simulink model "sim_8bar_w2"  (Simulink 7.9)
settings: Solver=ode45  StartTime=0.0  StopTime=10  RelTol=1e-3  AbsTol=1e-3
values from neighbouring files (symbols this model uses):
  g = 9806.65    [dyn_2dof.m]    (also in dyn_3dof.m; falling_sphere.m = 9.81; forward_2dof.m = 9.81)
  m = 1    [mechanical_system.m]
  s = Lv/norm(Lv)    [pkm1.m]
undefined symbols (not defined in the file or in its folder): cm, deg, kg, N
libraries: mblibv1 x55

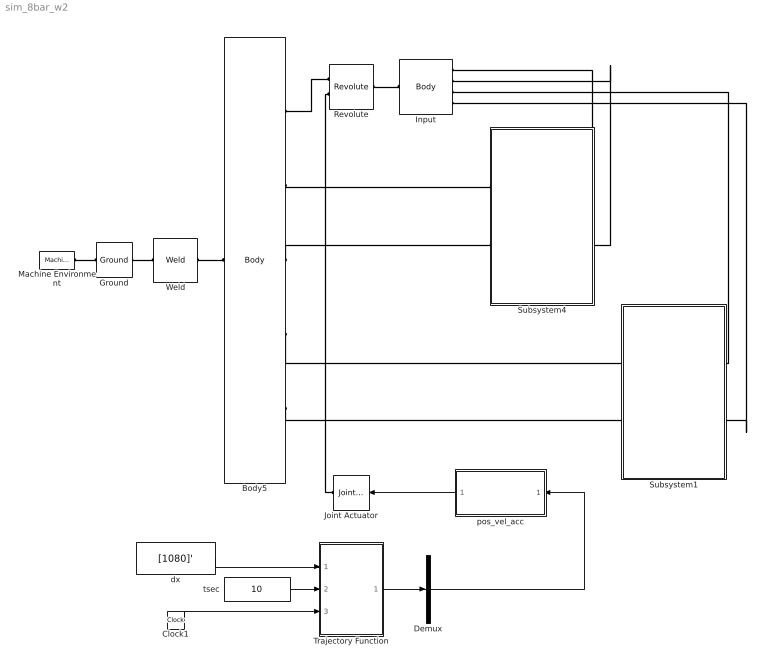
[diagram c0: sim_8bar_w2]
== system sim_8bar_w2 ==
  Body5 : mblibv1/Bodies/Body  LConnTagsString=CS1  RConnTagsString=CS2|CS3|CS4|CS5|CS6  UpdateFromCAD=off  DialogClass=MechanicalBodyBlock  Mass=50  MassUnits=g  InertiaUnits=g*cm^2  Inertia=[0 0 0; 0 0 0; 0 0 0]  Shape=Cylinder  ShapeDims=[1 1]  ShapeUnits=m  ShapeUse=false  Density=1  DensityUnits=kg/m^3  DensityUse=false  GraphicsMode=MACHINE_DEFAULT  BodyColorSelMode=MACHINE_DEFAULT  BodyColor=[1 0 0]  AttachedToCS=CG  CG=Left$CG$[0 0 0]$World$World$mm$[0 0 0]$Euler X-Y-Z$deg$WORLD$false$none  WorkingFrames=Left$CS1$[0 0 0]$World$World$mm$[0 0 0]$Euler X-Y-Z$deg$WORLD$true$none#Right$CS2$[0 0 0]$World$World$mm$[0 0 0]$Euler X-Y-Z$deg$WORLD$true$none#Right$CS3$[-52.5 0 0]$World$World$mm$[0 0 0]$Euler X-Y-Z$deg$WORLD$true$none#Right$CS4$[-52.5 0 0]$World$World$mm$[0 0 0]$Euler X-Y-Z$deg$WORLD$true$none#Right$CS5$[52.5 0 0]$World$World$mm$[0 0 0]$Euler X-Y-Z$deg$WORLD$true$none#Right$CS6$[52.5 0 0]$Worl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  CGPos=[0 0 0]  CGRot=[0 0 0]  CS0Pos=[]  CS0Rot=[]  CS1Pos=[0 0 0]  CS1Rot=[0 0 0]  CS2Pos=[0 0 0]  CS2Rot=[0 0 0]  CS3Pos=[-52.5 0 0]  CS3Rot=[0 0 0]  CS4Pos=[-52.5 0 0]  CS4Rot=[0 0 0]  CS5Pos=[52.5 0 0]  CS5Rot=[0 0 0]  CS6Pos=[52.5 0 0]  CS6Rot=[0 0 0]  CS7Pos=[]  CS7Rot=[]  CS8Pos=[]  CS8Rot=[]  CS9Pos=[]  CS9Rot=[]  CS10Pos=[]  CS10Rot=[]  CS11Pos=[]  CS11Rot=[]  CS12Pos=[]  CS12Rot=[]  CS13Pos=[]  CS13Rot=[]  CS14Pos=[]  CS14Rot=[]  CS15Pos=[]  CS15Rot=[]  CS16Pos=[]  CS16Rot=[]  CS17Pos=[]  CS17Rot=[]  CS18Pos=[]  CS18Rot=[]  CS19Pos=[]  CS19Rot=[]  CS20Pos=[]  CS20Rot=[]
  Clock1 : Clock
  Demux : Demux  Outputs=1
  Ground : mblibv1/Bodies/Ground  UpdateFromCAD=off  LeftPortType=env  RightPortType=workingframe  PhysicalDomain=Mechanical  DialogClass=GroundBlock  CoordPosition=[0 0 0]  CoordPositionUnits=mm  StateVectorMgrId=2  MachineId=[1 0]  ShowEnvPort=on
  Input : mblibv1/Bodies/Body  LConnTagsString=CS1  RConnTagsString=CS2|CS3|CS4|CS5  UpdateFromCAD=off  DialogClass=MechanicalBodyBlock  Mass=1.77  MassUnits=g  InertiaUnits=g*cm^2  Inertia=[1.2556 0 0; 0 1.2556 0; 0 0 0]  Shape=Cylinder  ShapeDims=[1 1]  ShapeUnits=m  ShapeUse=false  Density=1  DensityUnits=kg/m^3  DensityUse=false  GraphicsMode=MACHINE_DEFAULT  BodyColorSelMode=MACHINE_DEFAULT  BodyColor=[1 0 0]  AttachedToCS=CG  CG=Left$CG$[0 7.5 0]$CS1$CS1$mm$[0 0 0]$Euler X-Y-Z$deg$WORLD$false$none  WorkingFrames=Left$CS1$[0 0 0]$World$World$mm$[0 0 0]$Euler X-Y-Z$deg$WORLD$true$none#Right$CS2$[0 15 0]$World$World$mm$[0 0 0]$Euler X-Y-Z$deg$WORLD$true$none#Right$CS3$[0 15 0]$World$World$mm$[0 0 0]$Euler X-Y-Z$deg$WORLD$true$none#Right$CS4$[0 15 0]$World$World$mm$[0 0 0]$Euler X-Y-Z$deg$WORLD$true$none#Right$CS5$[0 15 0]$World$World$mm$[0 0 0]$Euler X-Y-Z$deg$WORLD$true$none  CGPos=[0 7.5 0]  CGRot=[0 0 0]  CS0Pos=[]  CS0Rot=[]  CS1Pos=[0 0 0]  CS1Rot=[0 0 0]  CS2Pos=[0 15 0]  CS2Rot=[0 0 0]  CS3Pos=[0 15 0]  CS3Rot=[0 0 0]  CS4Pos=[0 15 0]  CS4Rot=[0 0 0]  CS5Pos=[0 15 0]  CS5Rot=[0 0 0]  CS6Pos=[]  CS6Rot=[]  CS7Pos=[]  CS7Rot=[]  CS8Pos=[]  CS8Rot=[]  CS9Pos=[]  CS9Rot=[]  CS10Pos=[]  CS10Rot=[]  CS11Pos=[]  CS11Rot=[]  CS12Pos=[]  CS12Rot=[]  CS13Pos=[]  CS13Rot=[]  CS14Pos=[]  CS14Rot=[]  CS15Pos=[]  CS15Rot=[]  CS16Pos=[]  CS16Rot=[]  CS17Pos=[]  CS17Rot=[]  CS18Pos=[]  CS18Rot=[]  CS19Pos=[]  CS19Rot=[]  CS20Pos=[]  CS20Rot=[]
  Joint Actuator : mblibv1/Sensors &  Actuators/Joint Actuator  UpdateFromCAD=off  PhysicalDomain=Mechanical  PortType=blob  ActuationStyle=Motion  AngleUnits=deg  ArcVelocityUnits=deg/s  ArcAccelerationUnits=deg/s^2  CoordPositionUnits=m  VelocityUnits=m/s  AccelerationUnits=m/s^2  ForceUnits=N  TorqueUnits=N*m  ActiveIO=on  Width=3  DialogClass=MechanicalActuatorBlock  Primitive=R1  ReferenceFrame=Absolute (World)
  Machine Environment : mblibv1/Bodies/Machine Environment  PortType=env  PhysicalDomain=Mechanical  DialogTemplateClass=MECH.MachineEnvironment  SyncWhenCopied=off  Gravity=[0 -9.81 0]  GravityUnits=m/s^2  GravityAsSignal=off  Dimensionality=Auto-detect  AnalysisType=Forward dynamics  LinearAssemblyTolerance=1e-3  LinearAssemblyToleranceUnits=m  AngularAssemblyTolerance=1e-3  AngularAssemblyToleranceUnits=rad  ConstraintSolverType=Stabilizing  ConstraintRelTolerance=1e-4  ConstraintAbsTolerance=1e-4  UseRobustSingularityHandling=off  RedundancyAnalysisToleranceType=Automatically select tolerance  RedundancyAnalysisTolerance=1e-14  StatePerturbationType=Fixed  PerturbationSize=1e-5  VisualizeMachine=on  BodyVisualizationType=Use model default body geometries  BodyColorSelMode=Use model default  DefaultBodyColor=[1 0 0]
  Revolute : mblibv1/Joints/Revolute  LConnTagsString=__newl0|SA1  RConnTagsString=__newr0  UpdateFromCAD=off  NumSAPorts=1  CutJoint=off  MarkAsCut=off  Primitives=prismatic  PrimitiveProps=R1$World$[0 0 1]$revolute  DialogClass=JointBlock  R1Axis=[0 0 1]
  Subsystem1 : Subsystem
  Subsystem4 : Subsystem
  Trajectory Function : MATLAB Function  TreatAsAtomicUnit=on
  Weld : mblibv1/Joints/Weld  LConnTagsString=__newl0  RConnTagsString=__newr0  UpdateFromCAD=off  NumSAPorts=0  CutJoint=off  MarkAsCut=off  Primitives=weld  PrimitiveProps=W$WORLD$[0 0 0]$weld  DialogClass=JointBlock  WAxis=[0 0 0]
  dx : Constant  Value=[1080]'
  pos_vel_acc : Subsystem
  tsec : Constant  Value=10
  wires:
  Clock1/1 -> Trajectory Function/3(tout)
  tsec/1 -> Trajectory Function/2(tsec)
  dx/1 -> Trajectory Function/1(dx)
  Demux/1 -> pos_vel_acc/1(In1)
  Trajectory Function/1(xd) -> Demux/1
  pos_vel_acc/1(Motion1) -> Joint Actuator/1
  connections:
  Revolute/RConn1 -- Input/LConn1
  Subsystem4/LConn1 -- Input/RConn1
  Revolute/LConn1 -- Body5/RConn1
  Machine Environment/RConn1 -- Ground/LConn1
  Ground/RConn1 -- Weld/LConn1
  Weld/RConn1 -- Body5/LConn1
  Body5/RConn2 -- Subsystem4/RConn1
  Body5/RConn3 -- Subsystem4/RConn2
  Subsystem4/LConn2 -- Input/RConn2
  Joint Actuator/RConn1 -- Revolute/LConn2
  Body5/RConn4 -- Subsystem1/RConn1
  Body5/RConn5 -- Subsystem1/RConn2
  Input/RConn3 -- Subsystem1/LConn1
  Input/RConn4 -- Subsystem1/LConn2

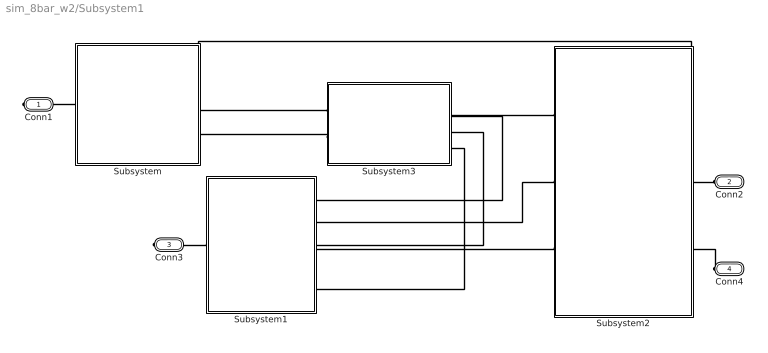
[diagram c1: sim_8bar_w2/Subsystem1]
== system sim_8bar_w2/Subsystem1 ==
  Subsystem : Subsystem
  Subsystem1 : Subsystem
  Subsystem2 : Subsystem
  Subsystem3 : Subsystem
  Conn1 : PMIOPort  Port=1  Side=Right
  Conn2 : PMIOPort  Port=2  Side=Left
  Conn3 : PMIOPort  Port=3  Side=Right
  Conn4 : PMIOPort  Port=4  Side=Left
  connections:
  Subsystem/LConn1 -- Subsystem2/LConn1
  Subsystem/LConn2 -- Subsystem3/LConn1
  Subsystem3/LConn2 -- Subsystem/LConn3
  Subsystem1/LConn1 -- Subsystem3/RConn2
  Subsystem1/LConn2 -- Subsystem2/RConn2
  Subsystem1/LConn3 -- Subsystem3/RConn3
  Subsystem1/LConn4 -- Subsystem2/RConn3
  Subsystem3/RConn4 -- Subsystem1/LConn5
  Subsystem3/RConn1 -- Subsystem2/RConn1
  Conn1/RConn1 -- Subsystem/RConn1
  Conn2/RConn1 -- Subsystem2/LConn2
  Conn3/RConn1 -- Subsystem1/RConn1
  Conn4/RConn1 -- Subsystem2/LConn3

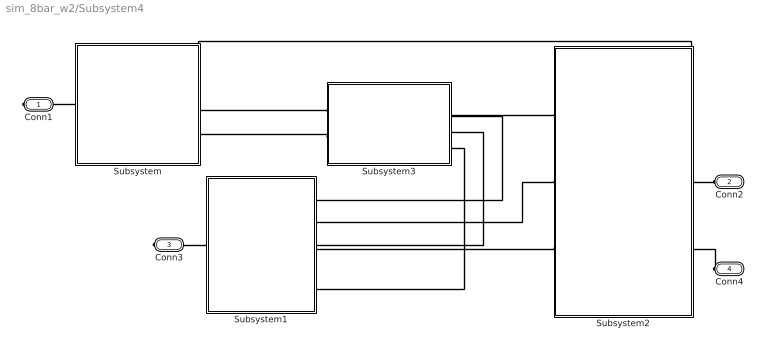
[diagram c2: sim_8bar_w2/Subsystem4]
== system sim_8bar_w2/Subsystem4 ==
  Subsystem : Subsystem
  Subsystem1 : Subsystem
  Subsystem2 : Subsystem
  Subsystem3 : Subsystem
  Conn1 : PMIOPort  Port=1  Side=Right
  Conn2 : PMIOPort  Port=2  Side=Left
  Conn3 : PMIOPort  Port=3  Side=Right
  Conn4 : PMIOPort  Port=4  Side=Left
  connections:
  Subsystem/LConn1 -- Subsystem2/LConn1
  Subsystem/LConn2 -- Subsystem3/LConn1
  Subsystem3/LConn2 -- Subsystem/LConn3
  Subsystem1/LConn1 -- Subsystem3/RConn2
  Subsystem1/LConn2 -- Subsystem2/RConn2
  Subsystem1/LConn3 -- Subsystem3/RConn3
  Subsystem1/LConn4 -- Subsystem2/RConn3
  Subsystem3/RConn4 -- Subsystem1/LConn5
  Subsystem3/RConn1 -- Subsystem2/RConn1
  Conn1/RConn1 -- Subsystem/RConn1
  Conn2/RConn1 -- Subsystem2/LConn2
  Conn3/RConn1 -- Subsystem1/RConn1
  Conn4/RConn1 -- Subsystem2/LConn3

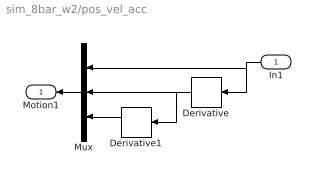
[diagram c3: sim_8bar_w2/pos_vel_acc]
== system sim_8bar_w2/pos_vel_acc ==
  In1 : Inport
  Derivative : Derivative
  Derivative1 : Derivative
  Mux : Mux  Inputs=3
  Motion1 : Outport
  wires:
  Derivative/1 -> Mux/2, Derivative1/1
  Derivative1/1 -> Mux/3
  In1/1 -> Mux/1, Derivative/1
  Mux/1 -> Motion1/1

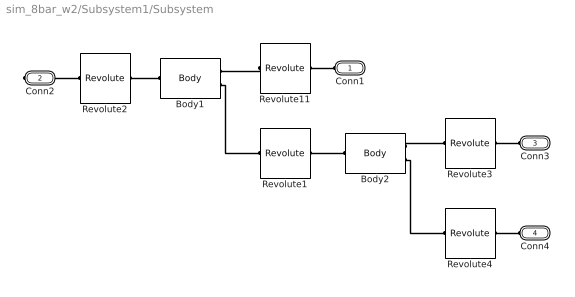
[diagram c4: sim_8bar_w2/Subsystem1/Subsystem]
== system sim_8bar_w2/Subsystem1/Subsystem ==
  Body1 : mblibv1/Bodies/Body  LConnTagsString=CS1  RConnTagsString=CS2|CS3  UpdateFromCAD=off  DialogClass=MechanicalBodyBlock  Mass=4.38  MassUnits=g  InertiaUnits=g*cm^2  Inertia=[4.1121 0 0; 0 4.1121 0; 0 0 0]  Shape=Cylinder  ShapeDims=[1 1]  ShapeUnits=m  ShapeUse=false  Density=1  DensityUnits=kg/m^3  DensityUse=false  GraphicsMode=MACHINE_DEFAULT  BodyColorSelMode=MACHINE_DEFAULT  BodyColor=[1 0 0]  AttachedToCS=CG  CG=Left$CG$[36.37/2 16.21/2 0]$CS1$CS1$mm$[0 0 0]$Euler X-Y-Z$deg$WORLD$false$none  WorkingFrames=Left$CS1$[52.5 0 0]$World$World$mm$[0 0 0]$Euler X-Y-Z$deg$WORLD$true$none#Right$CS2$[64.64 44.37 0]$World$World$mm$[0 0 0]$Euler X-Y-Z$deg$WORLD$true$none#Right$CS3$[96.87 -12.14 0]$World$World$mm$[0 0 0]$Euler X-Y-Z$deg$WORLD$true$none  CGPos=[36.37/2 16.21/2 0]  CGRot=[0 0 0]  CS0Pos=[]  CS0Rot=[]  CS1Pos=[52.5 0 0]  CS1Rot=[0 0 0]  CS2Pos=[64.64 44.37 0]  CS2Rot=[0 0 0]  CS3Pos=[96.87 -12.14 0]  CS3Rot=[0 0 0]  CS4Pos=[]  CS4Rot=[]  CS5Pos=[]  CS5Rot=[]  CS6Pos=[]  CS6Rot=[]  CS7Pos=[]  CS7Rot=[]  CS8Pos=[]  CS8Rot=[]  CS9Pos=[]  CS9Rot=[]  CS10Pos=[]  CS10Rot=[]  CS11Pos=[]  CS11Rot=[]  CS12Pos=[]  CS12Rot=[]  CS13Pos=[]  CS13Rot=[]  CS14Pos=[]  CS14Rot=[]  CS15Pos=[]  CS15Rot=[]  CS16Pos=[]  CS16Rot=[]  CS17Pos=[]  CS17Rot=[]  CS18Pos=[]  CS18Rot=[]  CS19Pos=[]  CS19Rot=[]  CS20Pos=[]  CS20Rot=[]
  Body2 : mblibv1/Bodies/Body  LConnTagsString=CS1  RConnTagsString=CS2|CS3  UpdateFromCAD=off  DialogClass=MechanicalBodyBlock  Mass=2.05  MassUnits=g  InertiaUnits=g*cm^2  Inertia=[1.1579 0 0; 0 1.1579 0; 0 0 0]  Shape=Cylinder  ShapeDims=[1 1]  ShapeUnits=m  ShapeUse=false  Density=1  DensityUnits=kg/m^3  DensityUse=false  GraphicsMode=MACHINE_DEFAULT  BodyColorSelMode=MACHINE_DEFAULT  BodyColor=[1 0 0]  AttachedToCS=CG  CG=Left$CG$[-13.02/2 -43.08/2 0]$CS1$CS1$mm$[0 0 0]$Euler X-Y-Z$deg$WORLD$false$none  WorkingFrames=Left$CS1$[96.87 -12.14 0]$World$World$mm$[0 0 0]$Euler X-Y-Z$deg$WORLD$true$none#Right$CS2$[83.85 -55.22 0]$World$World$mm$[0 0 0]$Euler X-Y-Z$deg$WORLD$true$none#Right$CS3$[83.85 -55.22 0]$World$World$mm$[0 0 0]$Euler X-Y-Z$deg$WORLD$true$none  CGPos=[-13.02/2 -43.08/2 0]  CGRot=[0 0 0]  CS0Pos=[]  CS0Rot=[]  CS1Pos=[96.87 -12.14 0]  CS1Rot=[0 0 0]  CS2Pos=[83.85 -55.22 0]  CS2Rot=[0 0 0]  CS3Pos=[83.85 -55.22 0]  CS3Rot=[0 0 0]  CS4Pos=[]  CS4Rot=[]  CS5Pos=[]  CS5Rot=[]  CS6Pos=[]  CS6Rot=[]  CS7Pos=[]  CS7Rot=[]  CS8Pos=[]  CS8Rot=[]  CS9Pos=[]  CS9Rot=[]  CS10Pos=[]  CS10Rot=[]  CS11Pos=[]  CS11Rot=[]  CS12Pos=[]  CS12Rot=[]  CS13Pos=[]  CS13Rot=[]  CS14Pos=[]  CS14Rot=[]  CS15Pos=[]  CS15Rot=[]  CS16Pos=[]  CS16Rot=[]  CS17Pos=[]  CS17Rot=[]  CS18Pos=[]  CS18Rot=[]  CS19Pos=[]  CS19Rot=[]  CS20Pos=[]  CS20Rot=[]
  Revolute{1..4,11} (5 alike) : mblibv1/Joints/Revolute  LConnTagsString=__newl0  RConnTagsString=__newr0  UpdateFromCAD=off  NumSAPorts=0  CutJoint=off  MarkAsCut=off  Primitives=prismatic  PrimitiveProps=R1$WORLD$[0 0 1]$revolute  DialogClass=JointBlock  R1Axis=[0 0 1]
  Conn1 : PMIOPort  Port=1  Side=Left
  Conn2 : PMIOPort  Port=2  Side=Right
  Conn3 : PMIOPort  Port=3  Side=Left
  Conn4 : PMIOPort  Port=4  Side=Left
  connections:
  Body1/LConn1 -- Revolute2/LConn1
  Revolute11/RConn1 -- Body1/RConn1
  Body1/RConn2 -- Revolute1/RConn1
  Revolute1/LConn1 -- Body2/LConn1
  Body2/RConn1 -- Revolute3/RConn1
  Body2/RConn2 -- Revolute4/RConn1
  Conn1/RConn1 -- Revolute11/LConn1
  Conn2/RConn1 -- Revolute2/RConn1
  Conn3/RConn1 -- Revolute3/LConn1
  Conn4/RConn1 -- Revolute4/LConn1

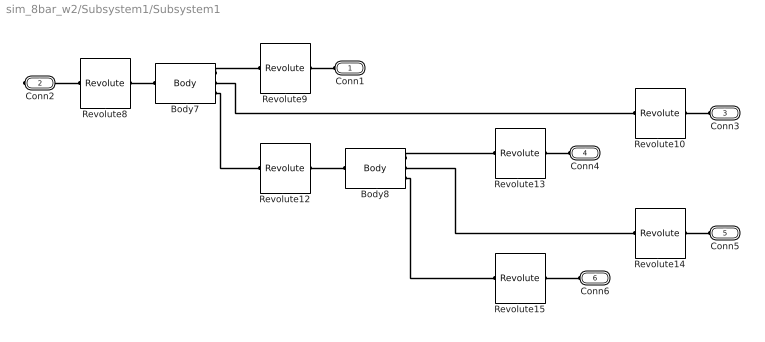
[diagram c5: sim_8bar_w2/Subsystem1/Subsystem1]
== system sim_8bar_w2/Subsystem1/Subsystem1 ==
  Body7 : mblibv1/Bodies/Body  LConnTagsString=CS1  RConnTagsString=CS2|CS3|CS4  UpdateFromCAD=off  DialogClass=MechanicalBodyBlock  Mass=7.25  MassUnits=g  InertiaUnits=g*cm^2  Inertia=[14.8828 0 0; 0 14.8828 0; 0 0 0]  Shape=Cylinder  ShapeDims=[1 1]  ShapeUnits=m  ShapeUse=false  Density=1  DensityUnits=kg/m^3  DensityUse=false  GraphicsMode=MACHINE_DEFAULT  BodyColorSelMode=MACHINE_DEFAULT  BodyColor=[1 0 0]  AttachedToCS=CG  CG=Left$CG$[-12.06/2 -43.55/2 0]$CS1$CS1$mm$[0 0 0]$Euler X-Y-Z$deg$WORLD$false$none  WorkingFrames=Left$CS1$[52.5 0 0]$World$World$mm$[0 0 0]$Euler X-Y-Z$deg$WORLD$true$none#Right$CS2$[40.44 -43.35 0]$World$World$mm$[0 0 0]$Euler X-Y-Z$deg$WORLD$true$none#Right$CS3$[40.44 -43.35 0]$World$World$mm$[0 0 0]$Euler X-Y-Z$deg$WORLD$true$none#Right$CS4$[40.44 -43.35 0]$World$World$mm$[0 0 0]$Euler X-Y-Z$deg$WORLD$true$none  CGPos=[-12.06/2 -43.55/2 0]  CGRot=[0 0 0]  CS0Pos=[]  CS0Rot=[]  CS1Pos=[52.5 0 0]  CS1Rot=[0 0 0]  CS2Pos=[40.44 -43.35 0]  CS2Rot=[0 0 0]  CS3Pos=[40.44 -43.35 0]  CS3Rot=[0 0 0]  CS4Pos=[40.44 -43.35 0]  CS4Rot=[0 0 0]  CS5Pos=[]  CS5Rot=[]  CS6Pos=[]  CS6Rot=[]  CS7Pos=[]  CS7Rot=[]  CS8Pos=[]  CS8Rot=[]  CS9Pos=[]  CS9Rot=[]  CS10Pos=[]  CS10Rot=[]  CS11Pos=[]  CS11Rot=[]  CS12Pos=[]  CS12Rot=[]  CS13Pos=[]  CS13Rot=[]  CS14Pos=[]  CS14Rot=[]  CS15Pos=[]  CS15Rot=[]  CS16Pos=[]  CS16Rot=[]  CS17Pos=[]  CS17Rot=[]  CS18Pos=[]  CS18Rot=[]  CS19Pos=[]  CS19Rot=[]  CS20Pos=[]  CS20Rot=[]
  Body8 : mblibv1/Bodies/Body  LConnTagsString=CS1  RConnTagsString=CS2|CS3|CS4  UpdateFromCAD=off  DialogClass=MechanicalBodyBlock  Mass=9.23  MassUnits=g  InertiaUnits=g*cm^2  Inertia=[7.7797 0 0; 0 7.7797 0; 0 0 0]  Shape=Cylinder  ShapeDims=[1 1]  ShapeUnits=m  ShapeUse=false  Density=1  DensityUnits=kg/m^3  DensityUse=false  GraphicsMode=MACHINE_DEFAULT  BodyColorSelMode=MACHINE_DEFAULT  BodyColor=[1 0 0]  AttachedToCS=CG  CG=Left$CG$[-16.47/2 -57.69/2 0]$CS1$CS1$mm$[0 0 0]$Euler X-Y-Z$deg$WORLD$false$none  WorkingFrames=Left$CS1$[40.44 -43.35 0]$World$World$mm$[0 0 0]$Euler X-Y-Z$deg$WORLD$true$none#Right$CS2$[40.44 -43.35 0]$World$World$mm$[0 0 0]$Euler X-Y-Z$deg$WORLD$true$none#Right$CS3$[40.44 -43.35 0]$World$World$mm$[0 0 0]$Euler X-Y-Z$deg$WORLD$true$none#Right$CS4$[28.09 -86.63 0]$World$World$mm$[0 0 0]$Euler X-Y-Z$deg$WORLD$true$none#Right$CS5$[23.97 -101.05 0]$World$World$mm$[0 0 0]$Euler X-Y-Z$deg$WORLD$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  CGPos=[-16.47/2 -57.69/2 0]  CGRot=[0 0 0]  CS0Pos=[]  CS0Rot=[]  CS1Pos=[40.44 -43.35 0]  CS1Rot=[0 0 0]  CS2Pos=[40.44 -43.35 0]  CS2Rot=[0 0 0]  CS3Pos=[40.44 -43.35 0]  CS3Rot=[0 0 0]  CS4Pos=[28.09 -86.63 0]  CS4Rot=[0 0 0]  CS5Pos=[23.97 -101.05 0]  CS5Rot=[0 0 0]  CS6Pos=[]  CS6Rot=[]  CS7Pos=[]  CS7Rot=[]  CS8Pos=[]  CS8Rot=[]  CS9Pos=[]  CS9Rot=[]  CS10Pos=[]  CS10Rot=[]  CS11Pos=[]  CS11Rot=[]  CS12Pos=[]  CS12Rot=[]  CS13Pos=[]  CS13Rot=[]  CS14Pos=[]  CS14Rot=[]  CS15Pos=[]  CS15Rot=[]  CS16Pos=[]  CS16Rot=[]  CS17Pos=[]  CS17Rot=[]  CS18Pos=[]  CS18Rot=[]  CS19Pos=[]  CS19Rot=[]  CS20Pos=[]  CS20Rot=[]
  Revolute{8..10,12..15} (7 alike) : mblibv1/Joints/Revolute  LConnTagsString=__newl0  RConnTagsString=__newr0  UpdateFromCAD=off  NumSAPorts=0  CutJoint=off  MarkAsCut=off  Primitives=prismatic  PrimitiveProps=R1$WORLD$[0 0 1]$revolute  DialogClass=JointBlock  R1Axis=[0 0 1]
  Conn1 : PMIOPort  Port=1  Side=Left
  Conn2 : PMIOPort  Port=2  Side=Right
  Conn3 : PMIOPort  Port=3  Side=Left
  Conn4 : PMIOPort  Port=4  Side=Left
  Conn5 : PMIOPort  Port=5  Side=Left
  Conn6 : PMIOPort  Port=6  Side=Left
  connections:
  Revolute8/LConn1 -- Body7/LConn1
  Body7/RConn1 -- Revolute9/RConn1
  Body7/RConn2 -- Revolute10/RConn1
  Body7/RConn3 -- Revolute12/RConn1
  Revolute12/LConn1 -- Body8/LConn1
  Body8/RConn1 -- Revolute13/RConn1
  Body8/RConn2 -- Revolute14/RConn1
  Body8/RConn3 -- Revolute15/RConn1
  Conn1/RConn1 -- Revolute9/LConn1
  Conn2/RConn1 -- Revolute8/RConn1
  Conn3/RConn1 -- Revolute10/LConn1
  Conn4/RConn1 -- Revolute13/LConn1
  Conn5/RConn1 -- Revolute14/LConn1
  Conn6/RConn1 -- Revolute15/LConn1

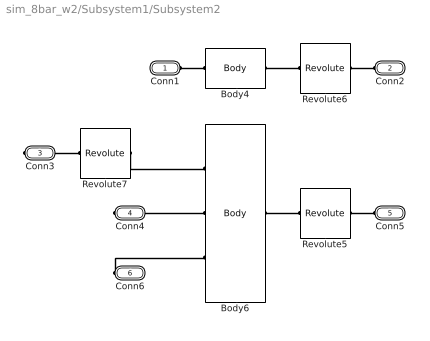
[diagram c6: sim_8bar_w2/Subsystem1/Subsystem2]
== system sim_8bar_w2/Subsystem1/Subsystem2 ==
  Body4 : mblibv1/Bodies/Body  LConnTagsString=CS1  RConnTagsString=CS2  UpdateFromCAD=off  DialogClass=MechanicalBodyBlock  Mass=2.27  MassUnits=g  InertiaUnits=g*cm^2  Inertia=[2.0686 0 0; 0 2.0686 0; 0 0 0]  Shape=Cylinder  ShapeDims=[1 1]  ShapeUnits=m  ShapeUse=false  Density=1  DensityUnits=kg/m^3  DensityUse=false  GraphicsMode=MACHINE_DEFAULT  BodyColorSelMode=MACHINE_DEFAULT  BodyColor=[1 0 0]  AttachedToCS=CG  CG=Left$CG$[-64.64/2 -29.37/2 0]$CS1$CS1$mm$[0 0 0]$Euler X-Y-Z$deg$WORLD$false$none  WorkingFrames=Left$CS1$[64.64 44.37 0]$World$World$mm$[0 0 0]$Euler X-Y-Z$deg$WORLD$true$none#Right$CS2$[0 15 0]$World$World$mm$[0 0 0]$Euler X-Y-Z$deg$WORLD$true$none  CGPos=[-64.64/2 -29.37/2 0]  CGRot=[0 0 0]  CS0Pos=[]  CS0Rot=[]  CS1Pos=[64.64 44.37 0]  CS1Rot=[0 0 0]  CS2Pos=[0 15 0]  CS2Rot=[0 0 0]  CS3Pos=[]  CS3Rot=[]  CS4Pos=[]  CS4Rot=[]  CS5Pos=[]  CS5Rot=[]  CS6Pos=[]  CS6Rot=[]  CS7Pos=[]  CS7Rot=[]  CS8Pos=[]  CS8Rot=[]  CS9Pos=[]  CS9Rot=[]  CS10Pos=[]  CS10Rot=[]  CS11Pos=[]  CS11Rot=[]  CS12Pos=[]  CS12Rot=[]  CS13Pos=[]  CS13Rot=[]  CS14Pos=[]  CS14Rot=[]  CS15Pos=[]  CS15Rot=[]  CS16Pos=[]  CS16Rot=[]  CS17Pos=[]  CS17Rot=[]  CS18Pos=[]  CS18Rot=[]  CS19Pos=[]  CS19Rot=[]  CS20Pos=[]  CS20Rot=[]
  Body6 : mblibv1/Bodies/Body  LConnTagsString=CS1  RConnTagsString=CS2|CS3|CS4  UpdateFromCAD=off  DialogClass=MechanicalBodyBlock  Mass=2.27  MassUnits=g  InertiaUnits=g*cm^2  Inertia=[2.0686 0 0; 0 2.0686 0; 0 0 0]  Shape=Cylinder  ShapeDims=[1 1]  ShapeUnits=m  ShapeUse=false  Density=1  DensityUnits=kg/m^3  DensityUse=false  GraphicsMode=MACHINE_DEFAULT  BodyColorSelMode=MACHINE_DEFAULT  BodyColor=[1 0 0]  AttachedToCS=CG  CG=Left$CG$[40.44/2 -58.35/2 0]$CS1$CS1$mm$[0 0 0]$Euler X-Y-Z$deg$WORLD$false$none  WorkingFrames=Left$CS1$[0 15 0]$World$World$mm$[0 0 0]$Euler X-Y-Z$deg$WORLD$true$none#Right$CS2$[40.44 -43.35 0]$World$World$mm$[0 0 0]$Euler X-Y-Z$deg$WORLD$true$none#Right$CS3$[40.44 -43.35 0]$World$World$mm$[0 0 0]$Euler X-Y-Z$deg$WORLD$true$none#Right$CS4$[40.44 -43.35 0]$World$World$mm$[0 0 0]$Euler X-Y-Z$deg$WORLD$true$none  CGPos=[40.44/2 -58.35/2 0]  CGRot=[0 0 0]  CS0Pos=[]  CS0Rot=[]  CS1Pos=[0 15 0]  CS1Rot=[0 0 0]  CS2Pos=[40.44 -43.35 0]  CS2Rot=[0 0 0]  CS3Pos=[40.44 -43.35 0]  CS3Rot=[0 0 0]  CS4Pos=[40.44 -43.35 0]  CS4Rot=[0 0 0]  CS5Pos=[]  CS5Rot=[]  CS6Pos=[]  CS6Rot=[]  CS7Pos=[]  CS7Rot=[]  CS8Pos=[]  CS8Rot=[]  CS9Pos=[]  CS9Rot=[]  CS10Pos=[]  CS10Rot=[]  CS11Pos=[]  CS11Rot=[]  CS12Pos=[]  CS12Rot=[]  CS13Pos=[]  CS13Rot=[]  CS14Pos=[]  CS14Rot=[]  CS15Pos=[]  CS15Rot=[]  CS16Pos=[]  CS16Rot=[]  CS17Pos=[]  CS17Rot=[]  CS18Pos=[]  CS18Rot=[]  CS19Pos=[]  CS19Rot=[]  CS20Pos=[]  CS20Rot=[]
  Revolute5 : mblibv1/Joints/Revolute  LConnTagsString=__newl0  RConnTagsString=__newr0  UpdateFromCAD=off  NumSAPorts=0  CutJoint=off  MarkAsCut=off  Primitives=prismatic  PrimitiveProps=R1$WORLD$[0 0 1]$revolute  DialogClass=JointBlock  R1Axis=[0 0 1]
  Revolute6 : mblibv1/Joints/Revolute  LConnTagsString=__newl0  RConnTagsString=__newr0  UpdateFromCAD=off  NumSAPorts=0  CutJoint=off  MarkAsCut=off  Primitives=prismatic  PrimitiveProps=R1$WORLD$[0 0 1]$revolute  DialogClass=JointBlock  R1Axis=[0 0 1]
  Revolute7 : mblibv1/Joints/Revolute  LConnTagsString=__newl0  RConnTagsString=__newr0  UpdateFromCAD=off  NumSAPorts=0  CutJoint=off  MarkAsCut=off  Primitives=prismatic  PrimitiveProps=R1$WORLD$[0 0 1]$revolute  DialogClass=JointBlock  R1Axis=[0 0 1]
  Conn1 : PMIOPort  Port=1  Side=Left
  Conn2 : PMIOPort  Port=2  Side=Left
  Conn3 : PMIOPort  Port=3  Side=Right
  Conn4 : PMIOPort  Port=4  Side=Right
  Conn5 : PMIOPort  Port=5  Side=Left
  Conn6 : PMIOPort  Port=6  Side=Right
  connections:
  Body4/RConn1 -- Revolute6/RConn1
  Body6/LConn1 -- Revolute5/RConn1
  Revolute7/LConn1 -- Body6/RConn1
  Conn1/RConn1 -- Body4/LConn1
  Conn2/RConn1 -- Revolute6/LConn1
  Conn3/RConn1 -- Revolute7/RConn1
  Conn4/RConn1 -- Body6/RConn2
  Conn5/RConn1 -- Revolute5/LConn1
  Conn6/RConn1 -- Body6/RConn3

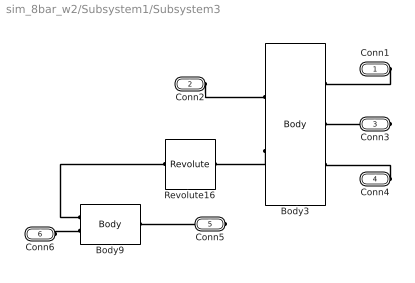
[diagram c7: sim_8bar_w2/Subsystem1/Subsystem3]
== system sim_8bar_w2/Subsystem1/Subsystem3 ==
  Body3 : mblibv1/Bodies/Body  LConnTagsString=CS1|CS5  RConnTagsString=CS2|CS3|CS4  UpdateFromCAD=off  DialogClass=MechanicalBodyBlock  Mass=2.05  MassUnits=g  InertiaUnits=g*cm^2  Inertia=[1.1579 0 0; 0 1.1579 0; 0 0 0]  Shape=Cylinder  ShapeDims=[1 1]  ShapeUnits=m  ShapeUse=false  Density=1  DensityUnits=kg/m^3  DensityUse=false  GraphicsMode=MACHINE_DEFAULT  BodyColorSelMode=MACHINE_DEFAULT  BodyColor=[1 0 0]  AttachedToCS=CG  CG=Left$CG$[-43.41/2 11.86/2 0]$CS1$CS1$mm$[0 0 0]$Euler X-Y-Z$deg$WORLD$false$none  WorkingFrames=Left$CS1$[83.85 -55.22 0]$World$World$mm$[0 0 0]$Euler X-Y-Z$deg$WORLD$true$none#Left$CS5$[83.85 -55.22 0]$World$World$mm$[0 0 0]$Euler X-Y-Z$deg$WORLD$true$none#Right$CS2$[40.44 -43.35 0]$World$World$mm$[0 0 0]$Euler X-Y-Z$deg$WORLD$true$none#Right$CS3$[40.44 -43.35 0]$World$World$mm$[0 0 0]$Euler X-Y-Z$deg$WORLD$true$none#Right$CS4$[40.44 -43.35 0]$World$World$mm$[0 0 0]$Euler X-Y-Z$deg$WORLD$tr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  CGPos=[-43.41/2 11.86/2 0]  CGRot=[0 0 0]  CS0Pos=[]  CS0Rot=[]  CS1Pos=[83.85 -55.22 0]  CS1Rot=[0 0 0]  CS2Pos=[40.44 -43.35 0]  CS2Rot=[0 0 0]  CS3Pos=[40.44 -43.35 0]  CS3Rot=[0 0 0]  CS4Pos=[40.44 -43.35 0]  CS4Rot=[0 0 0]  CS5Pos=[83.85 -55.22 0]  CS5Rot=[0 0 0]  CS6Pos=[]  CS6Rot=[]  CS7Pos=[]  CS7Rot=[]  CS8Pos=[]  CS8Rot=[]  CS9Pos=[]  CS9Rot=[]  CS10Pos=[]  CS10Rot=[]  CS11Pos=[]  CS11Rot=[]  CS12Pos=[]  CS12Rot=[]  CS13Pos=[]  CS13Rot=[]  CS14Pos=[]  CS14Rot=[]  CS15Pos=[]  CS15Rot=[]  CS16Pos=[]  CS16Rot=[]  CS17Pos=[]  CS17Rot=[]  CS18Pos=[]  CS18Rot=[]  CS19Pos=[]  CS19Rot=[]  CS20Pos=[]  CS20Rot=[]
  Body9 : mblibv1/Bodies/Body  LConnTagsString=CS1|CS2  RConnTagsString=CS3  UpdateFromCAD=off  DialogClass=MechanicalBodyBlock  Mass=2.85  MassUnits=g  InertiaUnits=g*cm^2  Inertia=[2.9339 0 0; 0 2.9339 0; 0 0 0]  Shape=Cylinder  ShapeDims=[1 1]  ShapeUnits=m  ShapeUse=false  Density=1  DensityUnits=kg/m^3  DensityUse=false  GraphicsMode=MACHINE_DEFAULT  BodyColorSelMode=MACHINE_DEFAULT  BodyColor=[1 0 0]  AttachedToCS=CG  CG=Left$CG$[-55.76/2 -31.41/2 0]$CS1$CS1$mm$[0 0 0]$Euler X-Y-Z$deg$WORLD$false$none  WorkingFrames=Left$CS1$[83.85 -55.22 0]$World$World$mm$[0 0 0]$Euler X-Y-Z$deg$WORLD$true$none#Left$CS2$[83.85 -55.22 0]$World$World$mm$[0 0 0]$Euler X-Y-Z$deg$WORLD$true$none#Right$CS3$[28.09 -86.63 0]$World$World$mm$[0 0 0]$Euler X-Y-Z$deg$WORLD$true$none  CGPos=[-55.76/2 -31.41/2 0]  CGRot=[0 0 0]  CS0Pos=[]  CS0Rot=[]  CS1Pos=[83.85 -55.22 0]  CS1Rot=[0 0 0]  CS2Pos=[83.85 -55.22 0]  CS2Rot=[0 0 0]  CS3Pos=[28.09 -86.63 0]  CS3Rot=[0 0 0]  CS4Pos=[]  CS4Rot=[]  CS5Pos=[]  CS5Rot=[]  CS6Pos=[]  CS6Rot=[]  CS7Pos=[]  CS7Rot=[]  CS8Pos=[]  CS8Rot=[]  CS9Pos=[]  CS9Rot=[]  CS10Pos=[]  CS10Rot=[]  CS11Pos=[]  CS11Rot=[]  CS12Pos=[]  CS12Rot=[]  CS13Pos=[]  CS13Rot=[]  CS14Pos=[]  CS14Rot=[]  CS15Pos=[]  CS15Rot=[]  CS16Pos=[]  CS16Rot=[]  CS17Pos=[]  CS17Rot=[]  CS18Pos=[]  CS18Rot=[]  CS19Pos=[]  CS19Rot=[]  CS20Pos=[]  CS20Rot=[]
  Revolute16 : mblibv1/Joints/Revolute  LConnTagsString=__newl0  RConnTagsString=__newr0  UpdateFromCAD=off  NumSAPorts=0  CutJoint=off  MarkAsCut=off  Primitives=prismatic  PrimitiveProps=R1$WORLD$[0 0 1]$revolute  DialogClass=JointBlock  R1Axis=[0 0 1]
  Conn1 : PMIOPort  Port=1  Side=Right
  Conn2 : PMIOPort  Port=2  Side=Left
  Conn3 : PMIOPort  Port=3  Side=Right
  Conn4 : PMIOPort  Port=4  Side=Right
  Conn5 : PMIOPort  Port=5  Side=Right
  Conn6 : PMIOPort  Port=6  Side=Left
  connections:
  Body3/LConn2 -- Revolute16/LConn1
  Body9/LConn1 -- Revolute16/RConn1
  Conn1/RConn1 -- Body3/RConn1
  Conn2/RConn1 -- Body3/LConn1
  Conn3/RConn1 -- Body3/RConn2
  Conn4/RConn1 -- Body3/RConn3
  Conn5/RConn1 -- Body9/RConn1
  Conn6/RConn1 -- Body9/LConn2

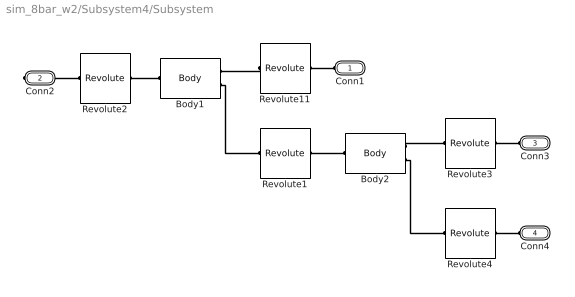
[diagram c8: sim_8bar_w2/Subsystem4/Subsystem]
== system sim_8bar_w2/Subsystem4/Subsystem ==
  Body1 : mblibv1/Bodies/Body  LConnTagsString=CS1  RConnTagsString=CS2|CS3  UpdateFromCAD=off  DialogClass=MechanicalBodyBlock  Mass=4.38  MassUnits=g  InertiaUnits=g*cm^2  Inertia=[4.1121 0 0; 0 4.1121 0; 0 0 0]  Shape=Cylinder  ShapeDims=[1 1]  ShapeUnits=m  ShapeUse=false  Density=1  DensityUnits=kg/m^3  DensityUse=false  GraphicsMode=MACHINE_DEFAULT  BodyColorSelMode=MACHINE_DEFAULT  BodyColor=[1 0 0]  AttachedToCS=CG  CG=Left$CG$[-36.37/2 16.21/2 0]$CS1$CS1$mm$[0 0 0]$Euler X-Y-Z$deg$WORLD$false$none  WorkingFrames=Left$CS1$[-52.5 0 0]$World$World$mm$[0 0 0]$Euler X-Y-Z$deg$WORLD$true$none#Right$CS2$[-64.64 44.37 0]$World$World$mm$[0 0 0]$Euler X-Y-Z$deg$WORLD$true$none#Right$CS3$[-96.87 -12.14 0]$World$World$mm$[0 0 0]$Euler X-Y-Z$deg$WORLD$true$none  CGPos=[-36.37/2 16.21/2 0]  CGRot=[0 0 0]  CS0Pos=[]  CS0Rot=[]  CS1Pos=[-52.5 0 0]  CS1Rot=[0 0 0]  CS2Pos=[-64.64 44.37 0]  CS2Rot=[0 0 0]  CS3Pos=[-96.87 -12.14 0]  CS3Rot=[0 0 0]  CS4Pos=[]  CS4Rot=[]  CS5Pos=[]  CS5Rot=[]  CS6Pos=[]  CS6Rot=[]  CS7Pos=[]  CS7Rot=[]  CS8Pos=[]  CS8Rot=[]  CS9Pos=[]  CS9Rot=[]  CS10Pos=[]  CS10Rot=[]  CS11Pos=[]  CS11Rot=[]  CS12Pos=[]  CS12Rot=[]  CS13Pos=[]  CS13Rot=[]  CS14Pos=[]  CS14Rot=[]  CS15Pos=[]  CS15Rot=[]  CS16Pos=[]  CS16Rot=[]  CS17Pos=[]  CS17Rot=[]  CS18Pos=[]  CS18Rot=[]  CS19Pos=[]  CS19Rot=[]  CS20Pos=[]  CS20Rot=[]
  Body2 : mblibv1/Bodies/Body  LConnTagsString=CS1  RConnTagsString=CS2|CS3  UpdateFromCAD=off  DialogClass=MechanicalBodyBlock  Mass=2.05  MassUnits=g  InertiaUnits=g*cm^2  Inertia=[1.1579 0 0; 0 1.1579 0; 0 0 0]  Shape=Cylinder  ShapeDims=[1 1]  ShapeUnits=m  ShapeUse=false  Density=1  DensityUnits=kg/m^3  DensityUse=false  GraphicsMode=MACHINE_DEFAULT  BodyColorSelMode=MACHINE_DEFAULT  BodyColor=[1 0 0]  AttachedToCS=CG  CG=Left$CG$[13.02/2 -43.08/2 0]$CS1$CS1$mm$[0 0 0]$Euler X-Y-Z$deg$WORLD$false$none  WorkingFrames=Left$CS1$[-96.87 -12.14 0]$World$World$mm$[0 0 0]$Euler X-Y-Z$deg$WORLD$true$none#Right$CS2$[-83.85 -55.22 0]$World$World$mm$[0 0 0]$Euler X-Y-Z$deg$WORLD$true$none#Right$CS3$[-83.85 -55.22 0]$World$World$mm$[0 0 0]$Euler X-Y-Z$deg$WORLD$true$none  CGPos=[13.02/2 -43.08/2 0]  CGRot=[0 0 0]  CS0Pos=[]  CS0Rot=[]  CS1Pos=[-96.87 -12.14 0]  CS1Rot=[0 0 0]  CS2Pos=[-83.85 -55.22 0]  CS2Rot=[0 0 0]  CS3Pos=[-83.85 -55.22 0]  CS3Rot=[0 0 0]  CS4Pos=[]  CS4Rot=[]  CS5Pos=[]  CS5Rot=[]  CS6Pos=[]  CS6Rot=[]  CS7Pos=[]  CS7Rot=[]  CS8Pos=[]  CS8Rot=[]  CS9Pos=[]  CS9Rot=[]  CS10Pos=[]  CS10Rot=[]  CS11Pos=[]  CS11Rot=[]  CS12Pos=[]  CS12Rot=[]  CS13Pos=[]  CS13Rot=[]  CS14Pos=[]  CS14Rot=[]  CS15Pos=[]  CS15Rot=[]  CS16Pos=[]  CS16Rot=[]  CS17Pos=[]  CS17Rot=[]  CS18Pos=[]  CS18Rot=[]  CS19Pos=[]  CS19Rot=[]  CS20Pos=[]  CS20Rot=[]
  Revolute{1..4,11} (5 alike) : mblibv1/Joints/Revolute  LConnTagsString=__newl0  RConnTagsString=__newr0  UpdateFromCAD=off  NumSAPorts=0  CutJoint=off  MarkAsCut=off  Primitives=prismatic  PrimitiveProps=R1$WORLD$[0 0 1]$revolute  DialogClass=JointBlock  R1Axis=[0 0 1]
  Conn1 : PMIOPort  Port=1  Side=Left
  Conn2 : PMIOPort  Port=2  Side=Right
  Conn3 : PMIOPort  Port=3  Side=Left
  Conn4 : PMIOPort  Port=4  Side=Left
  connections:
  Body1/LConn1 -- Revolute2/LConn1
  Revolute11/RConn1 -- Body1/RConn1
  Body1/RConn2 -- Revolute1/RConn1
  Revolute1/LConn1 -- Body2/LConn1
  Body2/RConn1 -- Revolute3/RConn1
  Body2/RConn2 -- Revolute4/RConn1
  Conn1/RConn1 -- Revolute11/LConn1
  Conn2/RConn1 -- Revolute2/RConn1
  Conn3/RConn1 -- Revolute3/LConn1
  Conn4/RConn1 -- Revolute4/LConn1

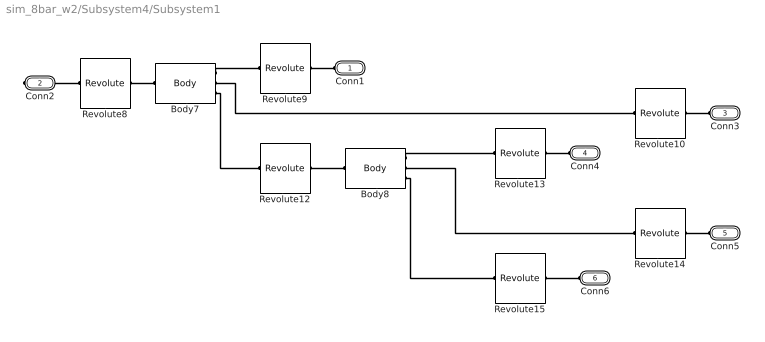
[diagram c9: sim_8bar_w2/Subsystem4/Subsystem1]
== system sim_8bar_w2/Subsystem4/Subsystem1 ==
  Body7 : mblibv1/Bodies/Body  LConnTagsString=CS1  RConnTagsString=CS2|CS3|CS4  UpdateFromCAD=off  DialogClass=MechanicalBodyBlock  Mass=7.25  MassUnits=g  InertiaUnits=g*cm^2  Inertia=[14.8828 0 0; 0 14.8828 0; 0 0 0]  Shape=Cylinder  ShapeDims=[1 1]  ShapeUnits=m  ShapeUse=false  Density=1  DensityUnits=kg/m^3  DensityUse=false  GraphicsMode=MACHINE_DEFAULT  BodyColorSelMode=MACHINE_DEFAULT  BodyColor=[1 0 0]  AttachedToCS=CG  CG=Left$CG$[12.06/2 -43.55/2 0]$CS1$CS1$mm$[0 0 0]$Euler X-Y-Z$deg$WORLD$false$none  WorkingFrames=Left$CS1$[-52.5 0 0]$World$World$mm$[0 0 0]$Euler X-Y-Z$deg$WORLD$true$none#Right$CS2$[-40.44 -43.35 0]$World$World$mm$[0 0 0]$Euler X-Y-Z$deg$WORLD$true$none#Right$CS3$[-40.44 -43.35 0]$World$World$mm$[0 0 0]$Euler X-Y-Z$deg$WORLD$true$none#Right$CS4$[-40.44 -43.35 0]$World$World$mm$[0 0 0]$Euler X-Y-Z$deg$WORLD$true$none  CGPos=[12.06/2 -43.55/2 0]  CGRot=[0 0 0]  CS0Pos=[]  CS0Rot=[]  CS1Pos=[-52.5 0 0]  CS1Rot=[0 0 0]  CS2Pos=[-40.44 -43.35 0]  CS2Rot=[0 0 0]  CS3Pos=[-40.44 -43.35 0]  CS3Rot=[0 0 0]  CS4Pos=[-40.44 -43.35 0]  CS4Rot=[0 0 0]  CS5Pos=[]  CS5Rot=[]  CS6Pos=[]  CS6Rot=[]  CS7Pos=[]  CS7Rot=[]  CS8Pos=[]  CS8Rot=[]  CS9Pos=[]  CS9Rot=[]  CS10Pos=[]  CS10Rot=[]  CS11Pos=[]  CS11Rot=[]  CS12Pos=[]  CS12Rot=[]  CS13Pos=[]  CS13Rot=[]  CS14Pos=[]  CS14Rot=[]  CS15Pos=[]  CS15Rot=[]  CS16Pos=[]  CS16Rot=[]  CS17Pos=[]  CS17Rot=[]  CS18Pos=[]  CS18Rot=[]  CS19Pos=[]  CS19Rot=[]  CS20Pos=[]  CS20Rot=[]
  Body8 : mblibv1/Bodies/Body  LConnTagsString=CS1  RConnTagsString=CS2|CS3|CS4  UpdateFromCAD=off  DialogClass=MechanicalBodyBlock  Mass=9.23  MassUnits=g  InertiaUnits=g*cm^2  Inertia=[7.7797 0 0; 0 7.7797 0; 0 0 0]  Shape=Cylinder  ShapeDims=[1 1]  ShapeUnits=m  ShapeUse=false  Density=1  DensityUnits=kg/m^3  DensityUse=false  GraphicsMode=MACHINE_DEFAULT  BodyColorSelMode=MACHINE_DEFAULT  BodyColor=[1 0 0]  AttachedToCS=CG  CG=Left$CG$[16.47/2 -57.69/2 0]$CS1$CS1$mm$[0 0 0]$Euler X-Y-Z$deg$WORLD$false$none  WorkingFrames=Left$CS1$[-40.44 -43.35 0]$World$World$mm$[0 0 0]$Euler X-Y-Z$deg$WORLD$true$none#Right$CS2$[-40.44 -43.35 0]$World$World$mm$[0 0 0]$Euler X-Y-Z$deg$WORLD$true$none#Right$CS3$[-40.44 -43.35 0]$World$World$mm$[0 0 0]$Euler X-Y-Z$deg$WORLD$true$none#Right$CS4$[-28.09 -86.63 0]$World$World$mm$[0 0 0]$Euler X-Y-Z$deg$WORLD$true$none#Right$CS5$[-23.97 -101.05 0]$World$World$mm$[0 0 0]$Euler X-Y-Z$deg$W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  CGPos=[16.47/2 -57.69/2 0]  CGRot=[0 0 0]  CS0Pos=[]  CS0Rot=[]  CS1Pos=[-40.44 -43.35 0]  CS1Rot=[0 0 0]  CS2Pos=[-40.44 -43.35 0]  CS2Rot=[0 0 0]  CS3Pos=[-40.44 -43.35 0]  CS3Rot=[0 0 0]  CS4Pos=[-28.09 -86.63 0]  CS4Rot=[0 0 0]  CS5Pos=[-23.97 -101.05 0]  CS5Rot=[0 0 0]  CS6Pos=[]  CS6Rot=[]  CS7Pos=[]  CS7Rot=[]  CS8Pos=[]  CS8Rot=[]  CS9Pos=[]  CS9Rot=[]  CS10Pos=[]  CS10Rot=[]  CS11Pos=[]  CS11Rot=[]  CS12Pos=[]  CS12Rot=[]  CS13Pos=[]  CS13Rot=[]  CS14Pos=[]  CS14Rot=[]  CS15Pos=[]  CS15Rot=[]  CS16Pos=[]  CS16Rot=[]  CS17Pos=[]  CS17Rot=[]  CS18Pos=[]  CS18Rot=[]  CS19Pos=[]  CS19Rot=[]  CS20Pos=[]  CS20Rot=[]
  Revolute{8..10,12..15} (7 alike) : mblibv1/Joints/Revolute  LConnTagsString=__newl0  RConnTagsString=__newr0  UpdateFromCAD=off  NumSAPorts=0  CutJoint=off  MarkAsCut=off  Primitives=prismatic  PrimitiveProps=R1$WORLD$[0 0 1]$revolute  DialogClass=JointBlock  R1Axis=[0 0 1]
  Conn1 : PMIOPort  Port=1  Side=Left
  Conn2 : PMIOPort  Port=2  Side=Right
  Conn3 : PMIOPort  Port=3  Side=Left
  Conn4 : PMIOPort  Port=4  Side=Left
  Conn5 : PMIOPort  Port=5  Side=Left
  Conn6 : PMIOPort  Port=6  Side=Left
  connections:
  Revolute8/LConn1 -- Body7/LConn1
  Body7/RConn1 -- Revolute9/RConn1
  Body7/RConn2 -- Revolute10/RConn1
  Body7/RConn3 -- Revolute12/RConn1
  Revolute12/LConn1 -- Body8/LConn1
  Body8/RConn1 -- Revolute13/RConn1
  Body8/RConn2 -- Revolute14/RConn1
  Body8/RConn3 -- Revolute15/RConn1
  Conn1/RConn1 -- Revolute9/LConn1
  Conn2/RConn1 -- Revolute8/RConn1
  Conn3/RConn1 -- Revolute10/LConn1
  Conn4/RConn1 -- Revolute13/LConn1
  Conn5/RConn1 -- Revolute14/LConn1
  Conn6/RConn1 -- Revolute15/LConn1

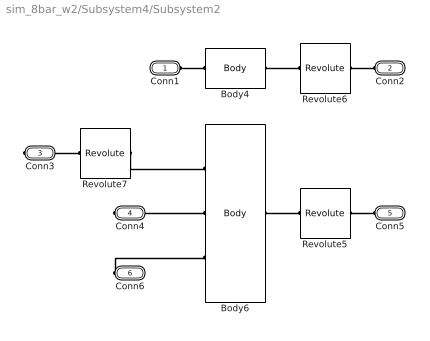
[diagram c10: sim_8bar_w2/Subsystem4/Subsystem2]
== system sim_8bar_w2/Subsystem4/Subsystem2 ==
  Body4 : mblibv1/Bodies/Body  LConnTagsString=CS1  RConnTagsString=CS2  UpdateFromCAD=off  DialogClass=MechanicalBodyBlock  Mass=2.27  MassUnits=g  InertiaUnits=g*cm^2  Inertia=[2.0686 0 0; 0 2.0686 0; 0 0 0]  Shape=Cylinder  ShapeDims=[1 1]  ShapeUnits=m  ShapeUse=false  Density=1  DensityUnits=kg/m^3  DensityUse=false  GraphicsMode=MACHINE_DEFAULT  BodyColorSelMode=MACHINE_DEFAULT  BodyColor=[1 0 0]  AttachedToCS=CG  CG=Left$CG$[64.64/2 -29.37/2 0]$CS1$CS1$mm$[0 0 0]$Euler X-Y-Z$deg$WORLD$false$none  WorkingFrames=Left$CS1$[-64.64 44.37 0]$World$World$mm$[0 0 0]$Euler X-Y-Z$deg$WORLD$true$none#Right$CS2$[0 15 0]$World$World$mm$[0 0 0]$Euler X-Y-Z$deg$WORLD$true$none  CGPos=[64.64/2 -29.37/2 0]  CGRot=[0 0 0]  CS0Pos=[]  CS0Rot=[]  CS1Pos=[-64.64 44.37 0]  CS1Rot=[0 0 0]  CS2Pos=[0 15 0]  CS2Rot=[0 0 0]  CS3Pos=[]  CS3Rot=[]  CS4Pos=[]  CS4Rot=[]  CS5Pos=[]  CS5Rot=[]  CS6Pos=[]  CS6Rot=[]  CS7Pos=[]  CS7Rot=[]  CS8Pos=[]  CS8Rot=[]  CS9Pos=[]  CS9Rot=[]  CS10Pos=[]  CS10Rot=[]  CS11Pos=[]  CS11Rot=[]  CS12Pos=[]  CS12Rot=[]  CS13Pos=[]  CS13Rot=[]  CS14Pos=[]  CS14Rot=[]  CS15Pos=[]  CS15Rot=[]  CS16Pos=[]  CS16Rot=[]  CS17Pos=[]  CS17Rot=[]  CS18Pos=[]  CS18Rot=[]  CS19Pos=[]  CS19Rot=[]  CS20Pos=[]  CS20Rot=[]
  Body6 : mblibv1/Bodies/Body  LConnTagsString=CS1  RConnTagsString=CS2|CS3|CS4  UpdateFromCAD=off  DialogClass=MechanicalBodyBlock  Mass=2.27  MassUnits=g  InertiaUnits=g*cm^2  Inertia=[2.0686 0 0; 0 2.0686 0; 0 0 0]  Shape=Cylinder  ShapeDims=[1 1]  ShapeUnits=m  ShapeUse=false  Density=1  DensityUnits=kg/m^3  DensityUse=false  GraphicsMode=MACHINE_DEFAULT  BodyColorSelMode=MACHINE_DEFAULT  BodyColor=[1 0 0]  AttachedToCS=CG  CG=Left$CG$[-40.44/2 -58.35/2 0]$CS1$CS1$mm$[0 0 0]$Euler X-Y-Z$deg$WORLD$false$none  WorkingFrames=Left$CS1$[0 15 0]$World$World$mm$[0 0 0]$Euler X-Y-Z$deg$WORLD$true$none#Right$CS2$[-40.44 -43.35 0]$World$World$mm$[0 0 0]$Euler X-Y-Z$deg$WORLD$true$none#Right$CS3$[-40.44 -43.35 0]$World$World$mm$[0 0 0]$Euler X-Y-Z$deg$WORLD$true$none#Right$CS4$[-40.44 -43.35 0]$World$World$mm$[0 0 0]$Euler X-Y-Z$deg$WORLD$true$none  CGPos=[-40.44/2 -58.35/2 0]  CGRot=[0 0 0]  CS0Pos=[]  CS0Rot=[]  CS1Pos=[0 15 0]  CS1Rot=[0 0 0]  CS2Pos=[-40.44 -43.35 0]  CS2Rot=[0 0 0]  CS3Pos=[-40.44 -43.35 0]  CS3Rot=[0 0 0]  CS4Pos=[-40.44 -43.35 0]  CS4Rot=[0 0 0]  CS5Pos=[]  CS5Rot=[]  CS6Pos=[]  CS6Rot=[]  CS7Pos=[]  CS7Rot=[]  CS8Pos=[]  CS8Rot=[]  CS9Pos=[]  CS9Rot=[]  CS10Pos=[]  CS10Rot=[]  CS11Pos=[]  CS11Rot=[]  CS12Pos=[]  CS12Rot=[]  CS13Pos=[]  CS13Rot=[]  CS14Pos=[]  CS14Rot=[]  CS15Pos=[]  CS15Rot=[]  CS16Pos=[]  CS16Rot=[]  CS17Pos=[]  CS17Rot=[]  CS18Pos=[]  CS18Rot=[]  CS19Pos=[]  CS19Rot=[]  CS20Pos=[]  CS20Rot=[]
  Revolute5 : mblibv1/Joints/Revolute  LConnTagsString=__newl0  RConnTagsString=__newr0  UpdateFromCAD=off  NumSAPorts=0  CutJoint=off  MarkAsCut=off  Primitives=prismatic  PrimitiveProps=R1$WORLD$[0 0 1]$revolute  DialogClass=JointBlock  R1Axis=[0 0 1]
  Revolute6 : mblibv1/Joints/Revolute  LConnTagsString=__newl0  RConnTagsString=__newr0  UpdateFromCAD=off  NumSAPorts=0  CutJoint=off  MarkAsCut=off  Primitives=prismatic  PrimitiveProps=R1$WORLD$[0 0 1]$revolute  DialogClass=JointBlock  R1Axis=[0 0 1]
  Revolute7 : mblibv1/Joints/Revolute  LConnTagsString=__newl0  RConnTagsString=__newr0  UpdateFromCAD=off  NumSAPorts=0  CutJoint=off  MarkAsCut=off  Primitives=prismatic  PrimitiveProps=R1$WORLD$[0 0 1]$revolute  DialogClass=JointBlock  R1Axis=[0 0 1]
  Conn1 : PMIOPort  Port=1  Side=Left
  Conn2 : PMIOPort  Port=2  Side=Left
  Conn3 : PMIOPort  Port=3  Side=Right
  Conn4 : PMIOPort  Port=4  Side=Right
  Conn5 : PMIOPort  Port=5  Side=Left
  Conn6 : PMIOPort  Port=6  Side=Right
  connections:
  Body4/RConn1 -- Revolute6/RConn1
  Body6/LConn1 -- Revolute5/RConn1
  Revolute7/LConn1 -- Body6/RConn1
  Conn1/RConn1 -- Body4/LConn1
  Conn2/RConn1 -- Revolute6/LConn1
  Conn3/RConn1 -- Revolute7/RConn1
  Conn4/RConn1 -- Body6/RConn2
  Conn5/RConn1 -- Revolute5/LConn1
  Conn6/RConn1 -- Body6/RConn3

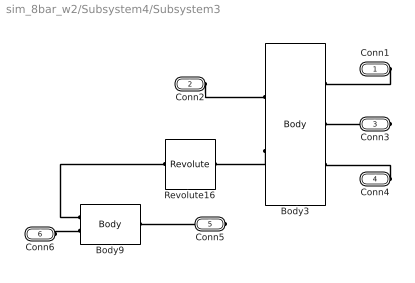
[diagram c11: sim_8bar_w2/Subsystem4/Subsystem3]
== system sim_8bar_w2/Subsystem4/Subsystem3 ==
  Body3 : mblibv1/Bodies/Body  LConnTagsString=CS1|CS5  RConnTagsString=CS2|CS3|CS4  UpdateFromCAD=off  DialogClass=MechanicalBodyBlock  Mass=2.05  MassUnits=g  InertiaUnits=g*cm^2  Inertia=[1.1579 0 0; 0 1.1579 0; 0 0 0]  Shape=Cylinder  ShapeDims=[1 1]  ShapeUnits=m  ShapeUse=false  Density=1  DensityUnits=kg/m^3  DensityUse=false  GraphicsMode=MACHINE_DEFAULT  BodyColorSelMode=MACHINE_DEFAULT  BodyColor=[1 0 0]  AttachedToCS=CG  CG=Left$CG$[43.41/2 11.86/2 0]$CS1$CS1$mm$[0 0 0]$Euler X-Y-Z$deg$WORLD$false$none  WorkingFrames=Left$CS1$[-83.85 -55.22 0]$World$World$mm$[0 0 0]$Euler X-Y-Z$deg$WORLD$true$none#Left$CS5$[-83.85 -55.22 0]$World$World$mm$[0 0 0]$Euler X-Y-Z$deg$WORLD$true$none#Right$CS2$[-40.44 -43.35 0]$World$World$mm$[0 0 0]$Euler X-Y-Z$deg$WORLD$true$none#Right$CS3$[-40.44 -43.35 0]$World$World$mm$[0 0 0]$Euler X-Y-Z$deg$WORLD$true$none#Right$CS4$[-40.44 -43.35 0]$World$World$mm$[0 0 0]$Euler X-Y-Z$deg$WOR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  CGPos=[43.41/2 11.86/2 0]  CGRot=[0 0 0]  CS0Pos=[]  CS0Rot=[]  CS1Pos=[-83.85 -55.22 0]  CS1Rot=[0 0 0]  CS2Pos=[-40.44 -43.35 0]  CS2Rot=[0 0 0]  CS3Pos=[-40.44 -43.35 0]  CS3Rot=[0 0 0]  CS4Pos=[-40.44 -43.35 0]  CS4Rot=[0 0 0]  CS5Pos=[-83.85 -55.22 0]  CS5Rot=[0 0 0]  CS6Pos=[]  CS6Rot=[]  CS7Pos=[]  CS7Rot=[]  CS8Pos=[]  CS8Rot=[]  CS9Pos=[]  CS9Rot=[]  CS10Pos=[]  CS10Rot=[]  CS11Pos=[]  CS11Rot=[]  CS12Pos=[]  CS12Rot=[]  CS13Pos=[]  CS13Rot=[]  CS14Pos=[]  CS14Rot=[]  CS15Pos=[]  CS15Rot=[]  CS16Pos=[]  CS16Rot=[]  CS17Pos=[]  CS17Rot=[]  CS18Pos=[]  CS18Rot=[]  CS19Pos=[]  CS19Rot=[]  CS20Pos=[]  CS20Rot=[]
  Body9 : mblibv1/Bodies/Body  LConnTagsString=CS1|CS2  RConnTagsString=CS3  UpdateFromCAD=off  DialogClass=MechanicalBodyBlock  Mass=2.85  MassUnits=g  InertiaUnits=g*cm^2  Inertia=[2.9339 0 0; 0 2.9339 0; 0 0 0]  Shape=Cylinder  ShapeDims=[1 1]  ShapeUnits=m  ShapeUse=false  Density=1  DensityUnits=kg/m^3  DensityUse=false  GraphicsMode=MACHINE_DEFAULT  BodyColorSelMode=MACHINE_DEFAULT  BodyColor=[1 0 0]  AttachedToCS=CG  CG=Left$CG$[55.76/2 -31.41/2 0]$CS1$CS1$mm$[0 0 0]$Euler X-Y-Z$deg$WORLD$false$none  WorkingFrames=Left$CS1$[-83.85 -55.22 0]$World$World$mm$[0 0 0]$Euler X-Y-Z$deg$WORLD$true$none#Left$CS2$[-83.85 -55.22 0]$World$World$mm$[0 0 0]$Euler X-Y-Z$deg$WORLD$true$none#Right$CS3$[-28.09 -86.63 0]$World$World$mm$[0 0 0]$Euler X-Y-Z$deg$WORLD$true$none  CGPos=[55.76/2 -31.41/2 0]  CGRot=[0 0 0]  CS0Pos=[]  CS0Rot=[]  CS1Pos=[-83.85 -55.22 0]  CS1Rot=[0 0 0]  CS2Pos=[-83.85 -55.22 0]  CS2Rot=[0 0 0]  CS3Pos=[-28.09 -86.63 0]  CS3Rot=[0 0 0]  CS4Pos=[]  CS4Rot=[]  CS5Pos=[]  CS5Rot=[]  CS6Pos=[]  CS6Rot=[]  CS7Pos=[]  CS7Rot=[]  CS8Pos=[]  CS8Rot=[]  CS9Pos=[]  CS9Rot=[]  CS10Pos=[]  CS10Rot=[]  CS11Pos=[]  CS11Rot=[]  CS12Pos=[]  CS12Rot=[]  CS13Pos=[]  CS13Rot=[]  CS14Pos=[]  CS14Rot=[]  CS15Pos=[]  CS15Rot=[]  CS16Pos=[]  CS16Rot=[]  CS17Pos=[]  CS17Rot=[]  CS18Pos=[]  CS18Rot=[]  CS19Pos=[]  CS19Rot=[]  CS20Pos=[]  CS20Rot=[]
  Revolute16 : mblibv1/Joints/Revolute  LConnTagsString=__newl0  RConnTagsString=__newr0  UpdateFromCAD=off  NumSAPorts=0  CutJoint=off  MarkAsCut=off  Primitives=prismatic  PrimitiveProps=R1$WORLD$[0 0 1]$revolute  DialogClass=JointBlock  R1Axis=[0 0 1]
  Conn1 : PMIOPort  Port=1  Side=Right
  Conn2 : PMIOPort  Port=2  Side=Left
  Conn3 : PMIOPort  Port=3  Side=Right
  Conn4 : PMIOPort  Port=4  Side=Right
  Conn5 : PMIOPort  Port=5  Side=Right
  Conn6 : PMIOPort  Port=6  Side=Left
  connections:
  Body3/LConn2 -- Revolute16/LConn1
  Body9/LConn1 -- Revolute16/RConn1
  Conn1/RConn1 -- Body3/RConn1
  Conn2/RConn1 -- Body3/LConn1
  Conn3/RConn1 -- Body3/RConn2
  Conn4/RConn1 -- Body3/RConn3
  Conn5/RConn1 -- Body9/RConn1
  Conn6/RConn1 -- Body9/LConn2

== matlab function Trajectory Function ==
function xd = fcn(dx, tsec, tout)

MAX_CH=1;       % Two Actuators %
D2R=pi/180;

% Initializing Variables %
xd=zeros(MAX_CH,1);
x0=D2R*[0,0]';



    [c] = coeff_3rd(x0, zeros(MAX_CH,1), x0+dx, zeros(MAX_CH,1), tsec);
    for ch=1:MAX_CH
        xd(ch,1)=c(ch,1)+c(ch,2)*tout+c(ch,3)*tout^2+c(ch,4)*tout^3;    
    end

function [c] = coeff_3rd(sp, sv, ep, ev, tsec)
MAX_CH=1;
c=zeros(MAX_CH,4);
for ch=1:MAX_CH
    c(ch,1)=sp(ch,1);
    c(ch,2)=sv(ch,1);
    c(ch,3)=(3.0*(ep(ch,1)-sp(ch,1))-(2.0*sv(ch,1)+ev(ch,1))*tsec)/(tsec*tsec);
    c(ch,4)=(-2.0*(ep(ch,1)-sp(ch,1))+(sv(ch,1)+ev(ch,1))*tsec)/(tsec*tsec*tsec);
end
